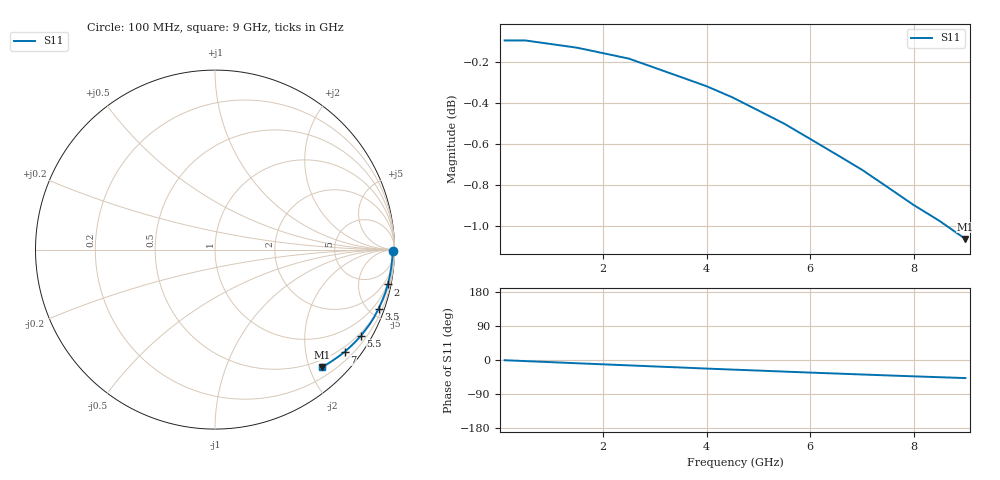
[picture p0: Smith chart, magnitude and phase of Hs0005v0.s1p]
!HSMS-0005 zero bias Schottky diode chip
!S-parameters at zero bias.  Last updated 6/7/94
# ghz s ma r 50
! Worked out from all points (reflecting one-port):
!   19 points, 100 MHz to 9 GHz, reference 50 ohm
!   lowest |S11| = -1.1 dB at 9 GHz (marker M1), VSWR 16.39, Z = 18.3 - j111 ohm
!   phase of S11 starts at -1 deg and turns -47 deg over the sweep
!   S11 on the Smith chart (normalised r, x): 100 MHz: open; 2 GHz: 0.91, -9.94; 3.5 GHz: 0.53, -5.68; 5.5 GHz: 0.41, -3.61; 7 GHz: 0.38, -2.84; 9 GHz: 0.37, -2.21
0.1  0.989 -0.6
0.5  0.989 -2.9
1  0.987 -5.7
1.5  0.985 -8.6
2  0.982 -11.4
2.5  0.979 -14.2
3  0.974 -17.0
3.5  0.969 -19.8
4  0.964 -22.6
4.5  0.958 -25.3
5  0.951 -27.9
5.5  0.944 -30.6
6  0.936 -33.2
6.5  0.928 -35.7
7  0.92 -38.2
7.5  0.911 -40.7
8  0.902 -43.1
8.5  0.894 -45.4
9  0.885 -47.7
